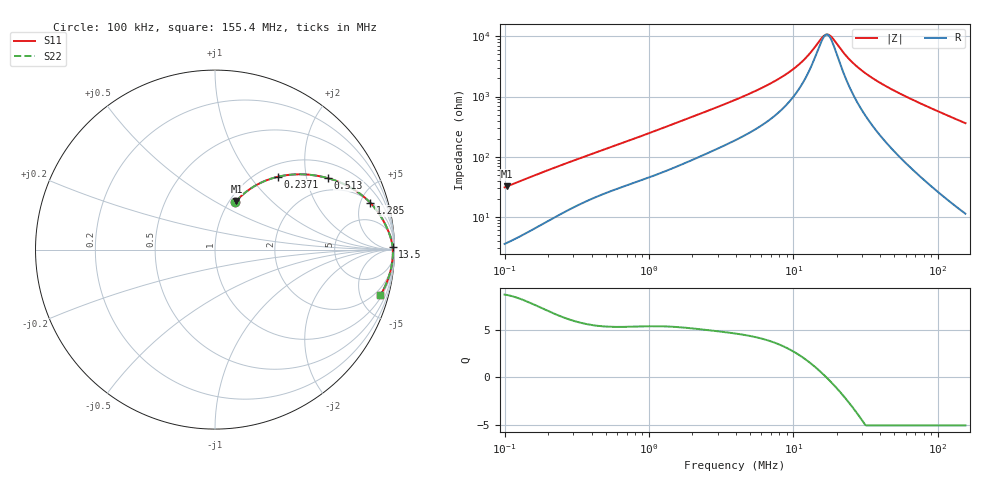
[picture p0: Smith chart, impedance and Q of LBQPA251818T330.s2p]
! LBQPA251818T330  S-PARAMETER MODEL  ( General Type )
! Model Generated by TAIYO YUDEN Corporation (http://www.ty-top.com)
! Version 1.0
! TAIYO YUDEN Control No. 191025NI43SB-FBB
! Copyright(c) 2019 TAIYO YUDEN CO.,LTD. All Rights Reserved.
! Product Description (link to TY-COMPAS)
! https://ds.yuden.co.jp/TYCOMPAS/or/detail?pn=LBQPA251818T330K&u=M
! Products Name : Inductors
! Characteristics :
!  Inductance : 33 uH , SRF(min) : 15 MHz , DC Resistance(max) : 1.95 Ohm
!  Rated Current : Saturation :270 mA , Temp Rise : 185 mA (20 degC)
!  Case Size : 2.5 x 1.8 / 0.098 x 0.071 [mm/inch] , Thickness : 1.8 / 0.071 [mm/inch]
!  (Conditions: Temperature = 25 degC , DC Bias Current/Voltage = 0A / 0V)
! External Node Assignments :
!  1  o---GGG---o  2
! GND o---------o GND
! Frequency Range : 0.1MHz  -  155.401204MHz  [ 402 STEP ]
# MHz S RI R 50
! Freq[MHz].  S11 Real  S11 Imag  S21 Real  S21 Imag  S12 Real  S12 Imag  S22 Real  S22 Imag
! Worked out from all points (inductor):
!   401 points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, 100 kHz to 155.4 MHz, reference 50 ohm
!   read as one part in series: L = 48.6 uH near 103.7 kHz
!   highest Q = 8.6 at 103.7 kHz (marker M1), where L = 49 uH
!   self-resonance near 16.83 MHz
!   S11 on the Smith chart (normalised r, x): 100 kHz: 1.07, +0.62; 237.1 kHz: 1.21, +1.38; 513 kHz: 1.51, +2.70; 1.285 MHz: 2.14, +6.07; 13.5 MHz: open; 155.4 MHz: 1.23, -7.22
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0.1  0.113 0.264  0.887 -0.264  0.887 -0.264  0.113 0.264
0.103743  0.1193 0.2712  0.8807 -0.2712  0.8807 -0.2712  0.1193 0.2712
0.152584  0.2069 0.3455  0.7931 -0.3455  0.7931 -0.3455  0.2069 0.3455
0.237135  0.3504 0.4059  0.6496 -0.4059  0.6496 -0.4059  0.3504 0.4059
0.342427  0.4866 0.4194  0.5134 -0.4194  0.5134 -0.4194  0.4866 0.4194
0.512978  0.6302 0.3976  0.3698 -0.3976  0.3698 -0.3976  0.6302 0.3976
1.172566  0.8496 0.2759  0.1504 -0.2759  0.1504 -0.2759  0.8496 0.2759
1.285377  0.8656 0.2599  0.1344 -0.2599  0.1344 -0.2599  0.8656 0.2599
2.110832  0.9268 0.18  0.0732 -0.18  0.0732 -0.18  0.9268 0.18
3.942096  0.965 0.1048  0.035 -0.1048  0.035 -0.1048  0.965 0.1048
6.126528  0.9788 0.0661  0.0212 -0.0661  0.0212 -0.0661  0.9788 0.0661
8.52766  0.985 0.0423  0.015 -0.0423  0.015 -0.0423  0.985 0.0423
11.02886  0.9881 0.0258  0.0119 -0.0258  0.0119 -0.0258  0.9881 0.0258
13.49882  0.9897 0.0136  0.0103 -0.0136  0.0103 -0.0136  0.9897 0.0136
16.22117  0.9906 0.00271  0.0094 -0.00271  0.0094 -0.00271  0.9906 0.00271
17.78178  0.9909 -0.00273  0.0091 0.00273  0.0091 0.00273  0.9909 -0.00273
23.42367  0.9912 -0.0195  0.00882 0.0195  0.00882 0.0195  0.9912 -0.0195
27.13214  0.9909 -0.029  0.00906 0.029  0.00906 0.029  0.9909 -0.029
34.45135  0.9899 -0.046  0.0101 0.046  0.0101 0.046  0.9899 -0.046
46.22367  0.9872 -0.0704  0.0128 0.0704  0.0128 0.0704  0.9872 -0.0704
80.20907  0.9739 -0.1333  0.0261 0.1333  0.0261 0.1333  0.9739 -0.1333
155.4012  0.922 -0.2529  0.078 0.2529  0.078 0.2529  0.922 -0.2529
